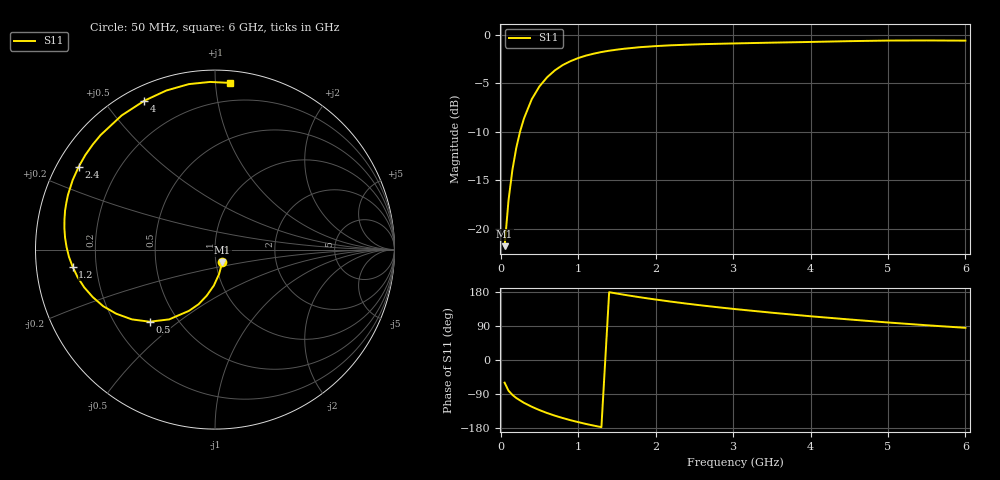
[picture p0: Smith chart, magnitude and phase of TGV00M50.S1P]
! SIEMENS Discrete & RF Semiconductors
! BAT64
! Si Schottky Diode in SOT23
! IF = 0.5 mA
! S-Parameters:  February  1997
# GHz  S  MA  R  50
!  f  S11
! GHz  MAG  ANG
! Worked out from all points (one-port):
!   34 points, 50 MHz to 6 GHz, reference 50 ohm
!   lowest |S11| = -21.8 dB at 50 MHz (marker M1), VSWR 1.18, Z = 53.7 - j7.62 ohm
!   |S11| at or under -10 dB: start of sweep to 248.8 MHz
!   S11 on the Smith chart (normalised r, x): 50 MHz: 1.07, -0.15; 500 MHz: 0.35, -0.40; 1.2 GHz: 0.11, -0.06; 2.4 GHz: 0.06, +0.28; 4 GHz: 0.06, +0.63; 6 GHz: 0.08, +1.09
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0.05  0.08153 -59.8
0.1  0.1398 -80.9
0.15  0.2006 -91.9
0.2  0.2608 -100.2
0.25  0.3177 -106.7
0.3  0.3706 -113.0
0.4  0.4652 -123.3
0.5  0.5423 -132.2
0.6  0.6048 -140.0
0.7  0.656 -147.0
0.8  0.698 -153.1
0.9  0.7308 -158.8
1  0.7585 -163.9
1.1  0.7808 -168.7
1.2  0.7989 -173.1
1.4  0.8275 178.9
1.6  0.8476 171.9
1.8  0.863 165.5
2  0.874 159.6
2.4  0.8887 148.8
2.6  0.8942 143.9
3  0.902 134.9
3.5  0.9106 124.8
4  0.9182 115.4
4.5  0.9269 107.0
5  0.9334 99.0
5.5  0.9346 91.7
6  0.9325 84.9
